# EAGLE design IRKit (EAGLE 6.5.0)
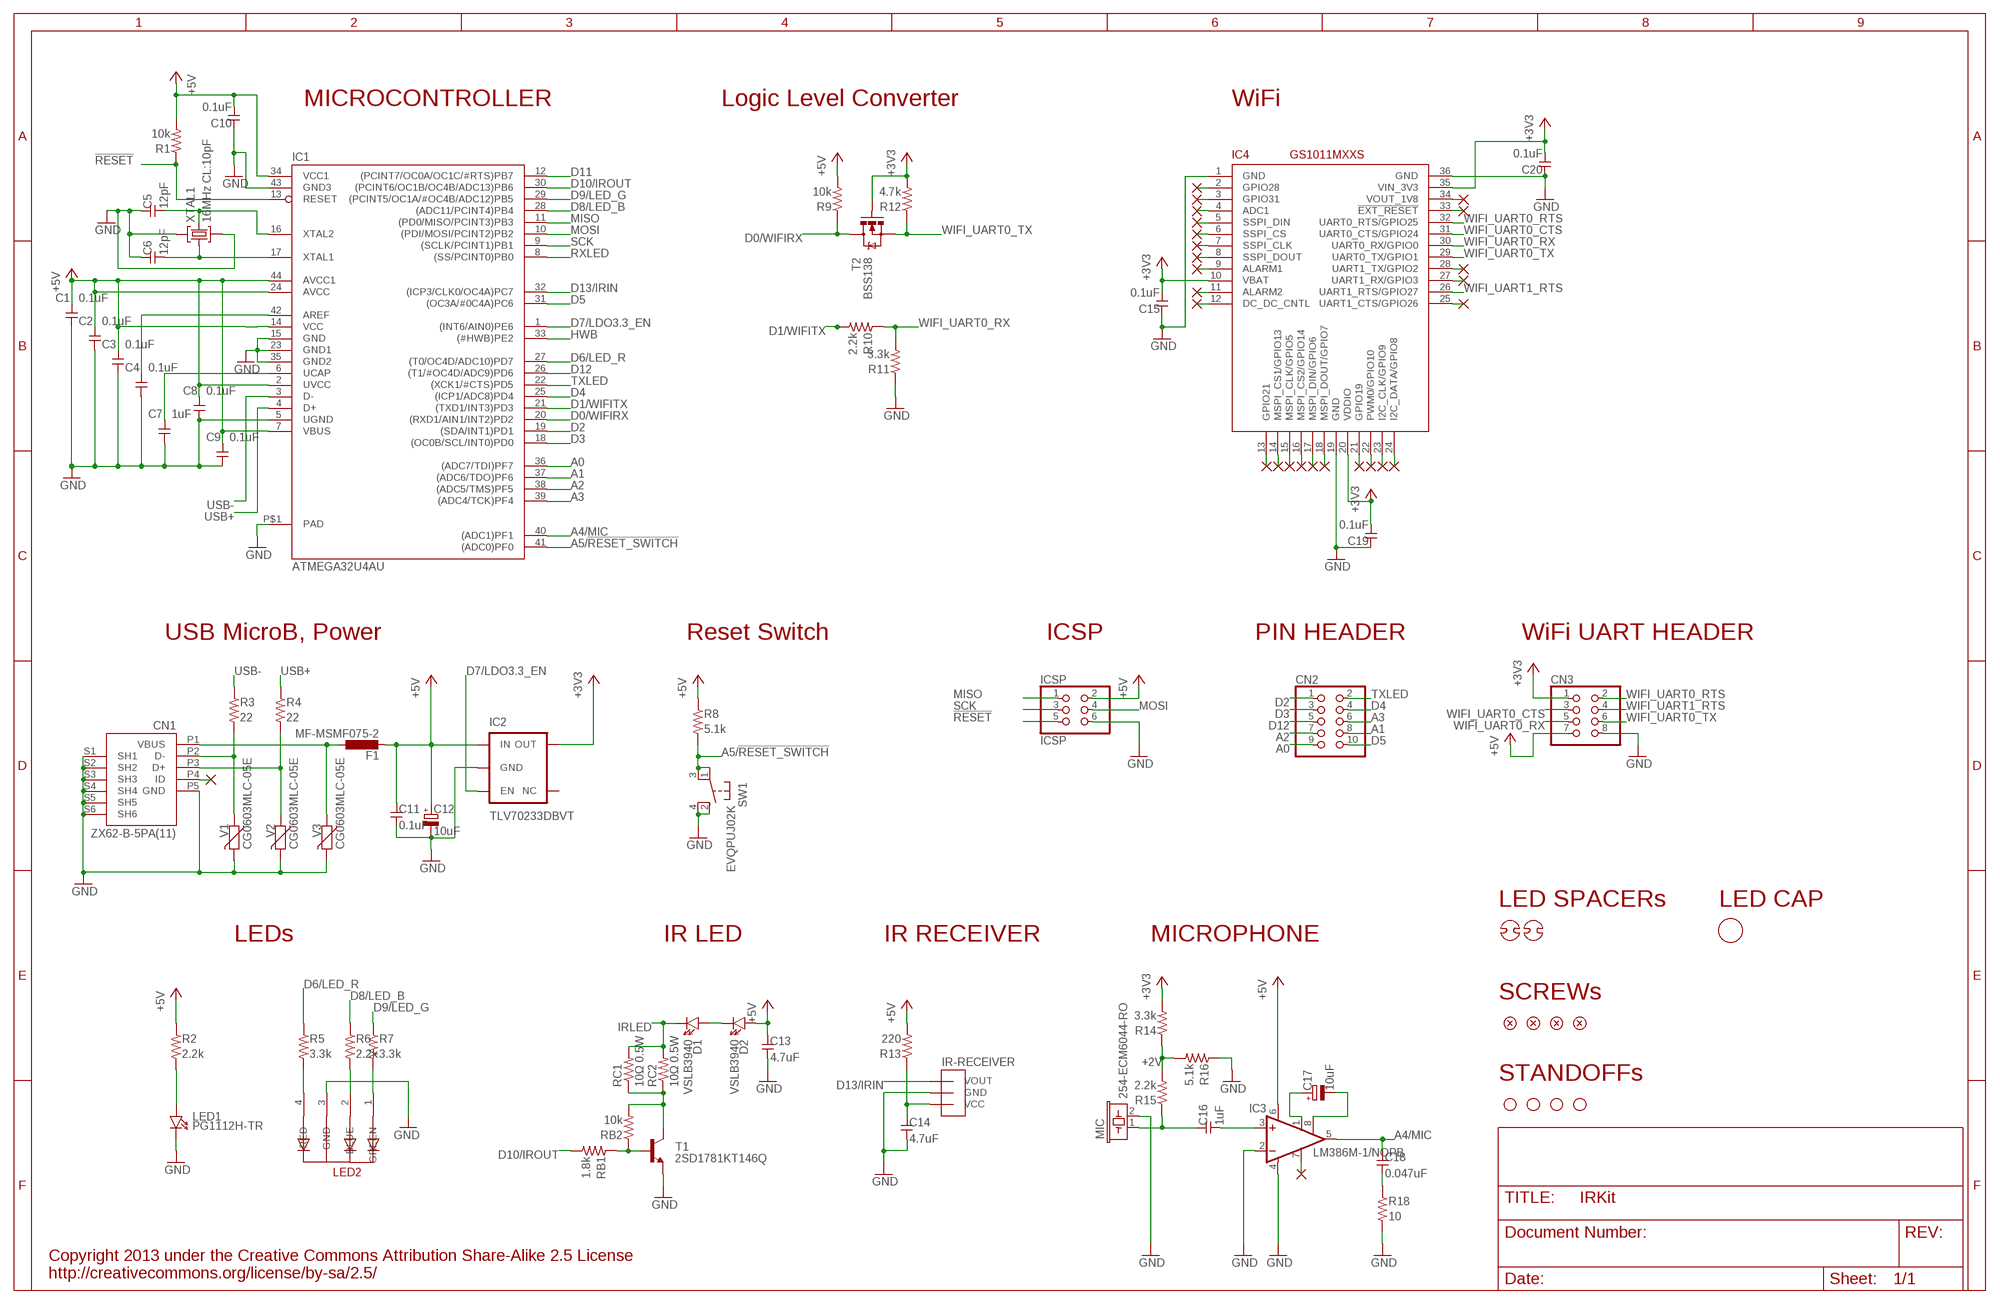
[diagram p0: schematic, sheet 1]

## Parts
C1  0.1uF  CAPACITOR2012  [SMD2012]
C2  0.1uF  CAPACITOR2012  [SMD2012]
C3  0.1uF  CAPACITOR2012  [SMD2012]
C4  0.1uF  CAPACITOR2012  [SMD2012]
C5  12pF  CAPACITOR2012  [SMD2012]
C6  12pF  CAPACITOR2012  [SMD2012]
C7  1uF  CAPACITOR2012  [SMD2012]
C8  0.1uF  CAPACITOR2012  [SMD2012]
C9  0.1uF  CAPACITOR2012  [SMD2012]
C10  0.1uF  CAPACITOR2012  [SMD2012]
C11  0.1uF  CAPACITOR2012  [SMD2012]
C12  10uF  CAPACITOR-POLPANASONIC_B  [PANASONIC_B]
C13  4.7uF  CAPACITOR2012  [SMD2012]
C14  4.7uF  CAPACITOR2012  [SMD2012]
C15  0.1uF  CAPACITOR2012  [SMD2012]
C16  1uF  CAPACITOR2012  [SMD2012]
C17  10uF  CAPACITOR-POLPANASONIC_B  [PANASONIC_B]
C18  0.047uF  CAPACITOR2012  [SMD2012]
C19  0.1uF  CAPACITOR2012  [SMD2012]
C20  0.1uF  CAPACITOR2012  [SMD2012]
CN1  ZX62-B-5PA(11)  USB-CONNECTORMICROB  [USB-MICROB]
CN2  PINHD-2X5  [2X05]
CN3  PINHD-2X4  [2X04]
D1  VSLB3940  LED-3MM  [LED3MM]
D2  VSLB3940  LED-3MM  [LED3MM]
F1  MF-MSMF075-2  L-EUL1812  [L1812]
IC1  ATMEGA32U4AU  [TQFP44-PAD]
IC2  TLV70233DBVT  TLV702XXSMD  [SOT23-5]
IC3  LM386M-1/NOPB  LM386M-1  [SO08]
IC4  GS1011MXXS  [GS1011MXXS]
ICSP  ICSP  PINHD-2X3  [2X03]
IR-RECEIVER  PL-IRM2161  [IR-RECEIVER]
LED1  PG1112H-TR  LED-2012  [LED2012]
LED2  5MMRGBLED  [LED5MMRGB]
LEDCAP1  LED-CAP  [LED-CAP]
MIC  254-ECM6044-RO  MICELECTRET_SMD  [MIC_SMD_4MM]
R1  10k  RESISTOR-US2012  [SMD2012]
R2  2.2k  RESISTOR-US2012  [SMD2012]
R3  22  RESISTOR-US2012  [SMD2012]
R4  22  RESISTOR-US2012  [SMD2012]
R5  3.3k  RESISTOR-US2012  [SMD2012]
R6  2.2k  RESISTOR-US2012  [SMD2012]
R7  3.3k  RESISTOR-US2012  [SMD2012]
R8  5.1k  RESISTOR-US2012  [SMD2012]
R9  10k  RESISTOR-US2012  [SMD2012]
R10  2.2k  RESISTOR-US2012  [SMD2012]
R11  3.3k  RESISTOR-US2012  [SMD2012]
R12  4.7k  RESISTOR-US2012  [SMD2012]
R13  220  RESISTOR-US2012  [SMD2012]
R14  3.3k  RESISTOR-US2012  [SMD2012]
R15  2.2k  RESISTOR-US2012  [SMD2012]
R16  5.1k  RESISTOR-US2012  [SMD2012]
R18  10  RESISTOR-US2012  [SMD2012]
RB1  1.8k  RESISTOR-US2012  [SMD2012]
RB2  10k  RESISTOR-US2012  [SMD2012]
RC1  10Ω 0.5W  R3225  [3225]
RC2  10Ω 0.5W  R3225  [3225]
SCREW1  flat-head M3 self-tapping  SCREW  [SCREW-M3]
SCREW2  flat-head M3 self-tapping  SCREW  [SCREW-M3]
SCREW3  flat-head M3 self-tapping  SCREW  [SCREW-M3]
SCREW4  flat-head M3 self-tapping  SCREW  [SCREW-M3]
SP1  LK-5  LED-SPACER-LK  [LED-SPACER-LK]
SP2  LK-5  LED-SPACER-LK  [LED-SPACER-LK]
STANDOFF1  STAND-OFF  [STAND-OFF]
STANDOFF2  STAND-OFF  [STAND-OFF]
STANDOFF3  STAND-OFF  [STAND-OFF]
STANDOFF4  STAND-OFF  [STAND-OFF]
SW1  EVQPUJ02K  TACTILE-SWITCHEVQPUJ02K  [TACTILE-SWITCH-EVQPUJ02K]
T1  2SD1781KT146Q  MMUN2211LT1-NPN-SC59-BEC  [SC59-BEC]
T2  BSS138  [SOT23]
V1  CG0603MLC-05E  VARISTORCN0603  [CT/CN0603]
V2  CG0603MLC-05E  VARISTORCN0603  [CT/CN0603]
V3  CG0603MLC-05E  VARISTORCN0603  [CT/CN0603]
XTAL1  16MHz CL:10pF  CRYSTAL-3.2-2.5  [CRYSTAL-3.2-2.5]

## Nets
!RESET: IC1.13(RESET) ICSP.5 R1.1
+2V: R14.1 R15.2 R16.2
+3V3 [3.3v]: C15.2 C19.2 C20.2 CN3.1 IC2.5(OUT) IC4.10(VBAT) IC4.20(VDDIO) IC4.35(VIN_3V3) R12.2 R14.2 T2.1(G)
+5V [power]: C1.2 C2.2 C3.2 C8.2 C9.2 C10.2 C11.1 C12.+ C13.1 CN3.7 D2.A F1.2 IC1.2(UVCC) IC1.7(VBUS) IC1.14(VCC) IC1.24(AVCC) IC1.34(VCC1) IC1.44(AVCC1) IC2.1(IN) IC3.6(VS) ICSP.2 R1.2 R2.1 R8.1 R9.2 R13.2
A0: CN2.9 IC1.36((ADC7/TDI)PF7)
A1: CN2.8 IC1.37((ADC6/TDO)PF6)
A2: CN2.7 IC1.38((ADC5/TMS)PF5)
A3: CN2.6 IC1.39((ADC4/TCK)PF4)
A4/MIC: C18.1 IC1.40((ADC1)PF1) IC3.5(OUT)
A5/!RESET_SWITCH: IC1.41((ADC0)PF0) R8.2 SW1.1(A) SW1.3(A)
AREF [power]: C4.2 IC1.42(AREF)
D0/WIFIRX: IC1.20((RXD1/AIN1/INT2)PD2) R9.1 T2.3(D)
D1/WIFITX: IC1.21((TXD1/INT3)PD3) R10.2
D2: CN2.1 IC1.19((SDA/INT1)PD1)
D3: CN2.3 IC1.18((OC0B/SCL/INT0)PD0)
D4: CN2.4 IC1.25((ICP1/ADC8)PD4)
D5: CN2.10 IC1.31((OC3A/#0C4A)PC6)
D6/LED_R: IC1.27((T0/OC4D/ADC10)PD7) R5.1
D7/LDO3.3_EN: IC1.1((INT6/AIN0)PE6) IC2.3(EN)
D8/LED_B: IC1.28((ADC11/PCINT4)PB4) R6.1
D9/LED_G: IC1.29((PCINT5/OC1A/#OC4B/ADC12)PB5) R7.1
D10/IROUT: IC1.30((PCINT6/OC1B/OC4B/ADC13)PB6) RB1.2
D11: IC1.12((PCINT7/OC0A/OC1C/#RTS)PB7)
D12: CN2.5 IC1.26((T1/#OC4D/ADC9)PD6)
D13/IRIN: IC1.32((ICP3/CLK0/OC4A)PC7) IR-RECEIVER.1(VOUT)
GND [gnd]: C1.1 C2.1 C3.1 C4.1 C5.1 C6.1 C7.1 C8.1 C9.1 C10.1 C11.2 C12.- C13.2 C14.2 C15.1 C19.1 C20.1 CN1.P5(GND) CN1.S1(SH1) CN1.S2(SH2) CN1.S3(SH3) CN1.S4(SH4) CN1.S5(SH5) CN1.S6(SH6) CN3.8 IC1.5(UGND) IC1.15(GND) IC1.23(GND1) IC1.35(GND2) IC1.43(GND3) IC1.P$1(PAD) IC2.2(GND) IC3.2(-IN) IC3.4(GND) IC4.1(GND) IC4.19(GND) IC4.36(GND) ICSP.6 IR-RECEIVER.2(GND) LED1.K LED2.3(GND) MIC.2 R11.1 R16.1 R18.2 SW1.2(B) SW1.4(B) T1.E V1.2 V2.2 V3.2 XTAL1.2(GND) XTAL1.4(GND)
HWB: IC1.33((#HWB)PE2)
IRLED [ir-power]: D1.K RC1.2 RC2.2
MICOUT: C16.1 MIC.1 R15.1
MISO: IC1.11((PD0/MISO/PCINT3)PB3) ICSP.1
MOSI: IC1.10((PDI/MOSI/PCINT2)PB2) ICSP.4
N$1: C17.- IC3.8(GAIN)
N$3: LED1.A R2.2
N$4: C16.2 IC3.3(+IN)
N$5: LED2.1(GREEN) R7.2
N$6: IC3.7(BYPASS)
N$8: C17.+ IC3.1(GAIN)
N$10: RB1.1 RB2.1 T1.B
N$11 [ir-power]: RB2.2 RC1.1 RC2.1 T1.C
N$14: C18.2 R18.1
N$16: C14.1 IR-RECEIVER.3(VCC) R13.1
N$17: LED2.2(BLUE) R6.2
N$18: IC4.2(GPIO28)
N$19: IC4.8(SSPI_DOUT)
N$20: IC4.9(ALARM1)
N$21: IC4.3(GPIO31)
N$22: IC4.4(ADC1)
N$23: IC4.5(SSPI_DIN)
N$24: IC4.6(SSPI_CS)
N$25: IC4.7(SSPI_CLK)
N$26: IC4.11(ALARM2)
N$27: IC4.12(DC_DC_CNTL)
N$28: IC4.13(GPIO21)
N$29: IC4.14(MSPI_CS1/GPIO13)
N$30: IC4.15(MSPI_CLK/GPIO5)
N$31: IC4.16(MSPI_CS2/GPIO14)
N$32: IC4.17(MSPI_DIN/GPIO6)
N$33: IC4.18(MSPI_DOUT/GPIO7)
N$34: IC4.21(GPIO19)
N$35: IC4.22(PWM0/GPIO10)
N$36: IC4.23(I2C_CLK/GPIO9)
N$37: IC4.24(I2C_DATA/GPIO8)
N$38: IC4.25(UART1_CTS/GPIO26)
N$39: IC4.27(UART1_RX/GPIO3)
N$40: IC4.28(UART1_TX/GPIO2)
N$41: LED2.4(RED) R5.2
N$43: IC4.34(VOUT_1V8)
N$44: IC4.33(!EXT_RESET)
N$48: CN1.P2(D-) R3.2 V1.1
N$51: CN1.P3(D+) R4.2 V2.1
N$52: CN1.P1(VBUS) F1.1 V3.1
N$58 [power]: D1.A D2.K
RXLED: IC1.8((SS/PCINT0)PB0)
SCK: IC1.9((SCLK/PCINT1)PB1) ICSP.3
TXLED: CN2.2 IC1.22((XCK1/#CTS)PD5)
UCAP: C7.2 IC1.6(UCAP)
USB+: IC1.4(D+) R4.1
USB-: IC1.3(D-) R3.1
USB-ID: CN1.P4(ID)
WIFI_UART0_CTS: CN3.3 IC4.31(UART0_CTS/GPIO24)
WIFI_UART0_RTS: CN3.2 IC4.32(UART0_RTS/GPIO25)
WIFI_UART0_RX: CN3.5 IC4.30(UART0_RX/GPIO0) R10.1 R11.2
WIFI_UART0_TX: CN3.6 IC4.29(UART0_TX/GPIO1) R12.1 T2.2(S)
WIFI_UART1_RTS: CN3.4 IC4.26(UART1_RTS/GPIO27)
XTAL1: C6.2 IC1.17(XTAL1) XTAL1.1(C1)
XTAL2: C5.2 IC1.16(XTAL2) XTAL1.3(C2)
Unconnected: IC2.4(NC)

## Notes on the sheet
- MICROCONTROLLER | Logic Level Converter | WiFi
- USB MicroB, Power | Reset Switch | ICSP | PIN HEADER | WiFi UART HEADER
- LED SPACERs | LED CAP
- LEDs | IR LED | IR RECEIVER | MICROPHONE
- SCREWs
- STANDOFFs
- Copyright 2013 under the Creative Commons Attribution Share-Alike 2.5 License
  http://creativecommons.org/license/by-sa/2.5/

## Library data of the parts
C1-C11 C13-C16 C18-C20 = my:CAPACITOR: Generic Capacitor
C12 C17 = my:CAPACITOR-POL: Generic Capacitor with Polarity
CN1 = my:USB-CONNECTOR
CN2 = my:PINHD-2X5: PIN HEADER
CN3 = my:PINHD-2X4: PIN HEADER
D1 D2 LED1 = my:LED: Through-hole LED
F1 = my:L-EU: INDUCTOR, European symbol
IC1 = my:ATMEGA32U4
IC2 = my:TLV702XX: TLV702xx http://www.tij.co.jp/jp/lit/ds/symlink/tlv70233.pdf http://www.ti.com/lit/ds/slvsag6b/slvsag6b.pdf 300-mA, Low-IQ, Low-Dropout Regulator
IC3 = my:LM386?-*: Low Voltage Audio Power Amplifier Source: http://cache.national.com/ds/LM/LM386.pdf
IC4 = my:GS1011MXXS
ICSP = my:PINHD-2X3: PIN HEADER
IR-RECEIVER = my:PL-IRM2161: PL-IRM2161-XD1 IR Receiver http://akizukidenshi.com/catalog/g/gI-06491/ http://akizukidenshi.com/download/ds/paralight/PL-IRM2161-XD1.pdf
LED2 = my:5MMRGBLED
LEDCAP1 = my:LED-CAP
MIC = my:MIC: Omni-directional electret condenser microphone.
R1-R16 R18 RB1 RB2 = my:RESISTOR-US: Generic Registor
RC1 RC2 = my:R: RESISTOR
SCREW1-SCREW4 = my:SCREW
SP1 SP2 = my:LED-SPACER
STANDOFF1-STANDOFF4 = my:STAND-OFF: #4 Stand Off
SW1 = my:TACTILE-SWITCH: TACTILE SWITCH
T1 = transistor:*-NPN-: NPN Transistror BF959 corrected 2008.03.06
T2 = my:BSS138
V1-V3 = my:VARISTOR: VARISTOR
XTAL1 = my:CRYSTAL-3.2-2.5

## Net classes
0 default: width 0.254 mm
1 power: width 0.406 mm
2 ir-power: width 0.813 mm
3 gnd: width 0.406 mm
4 3.3v: width 0.406 mm

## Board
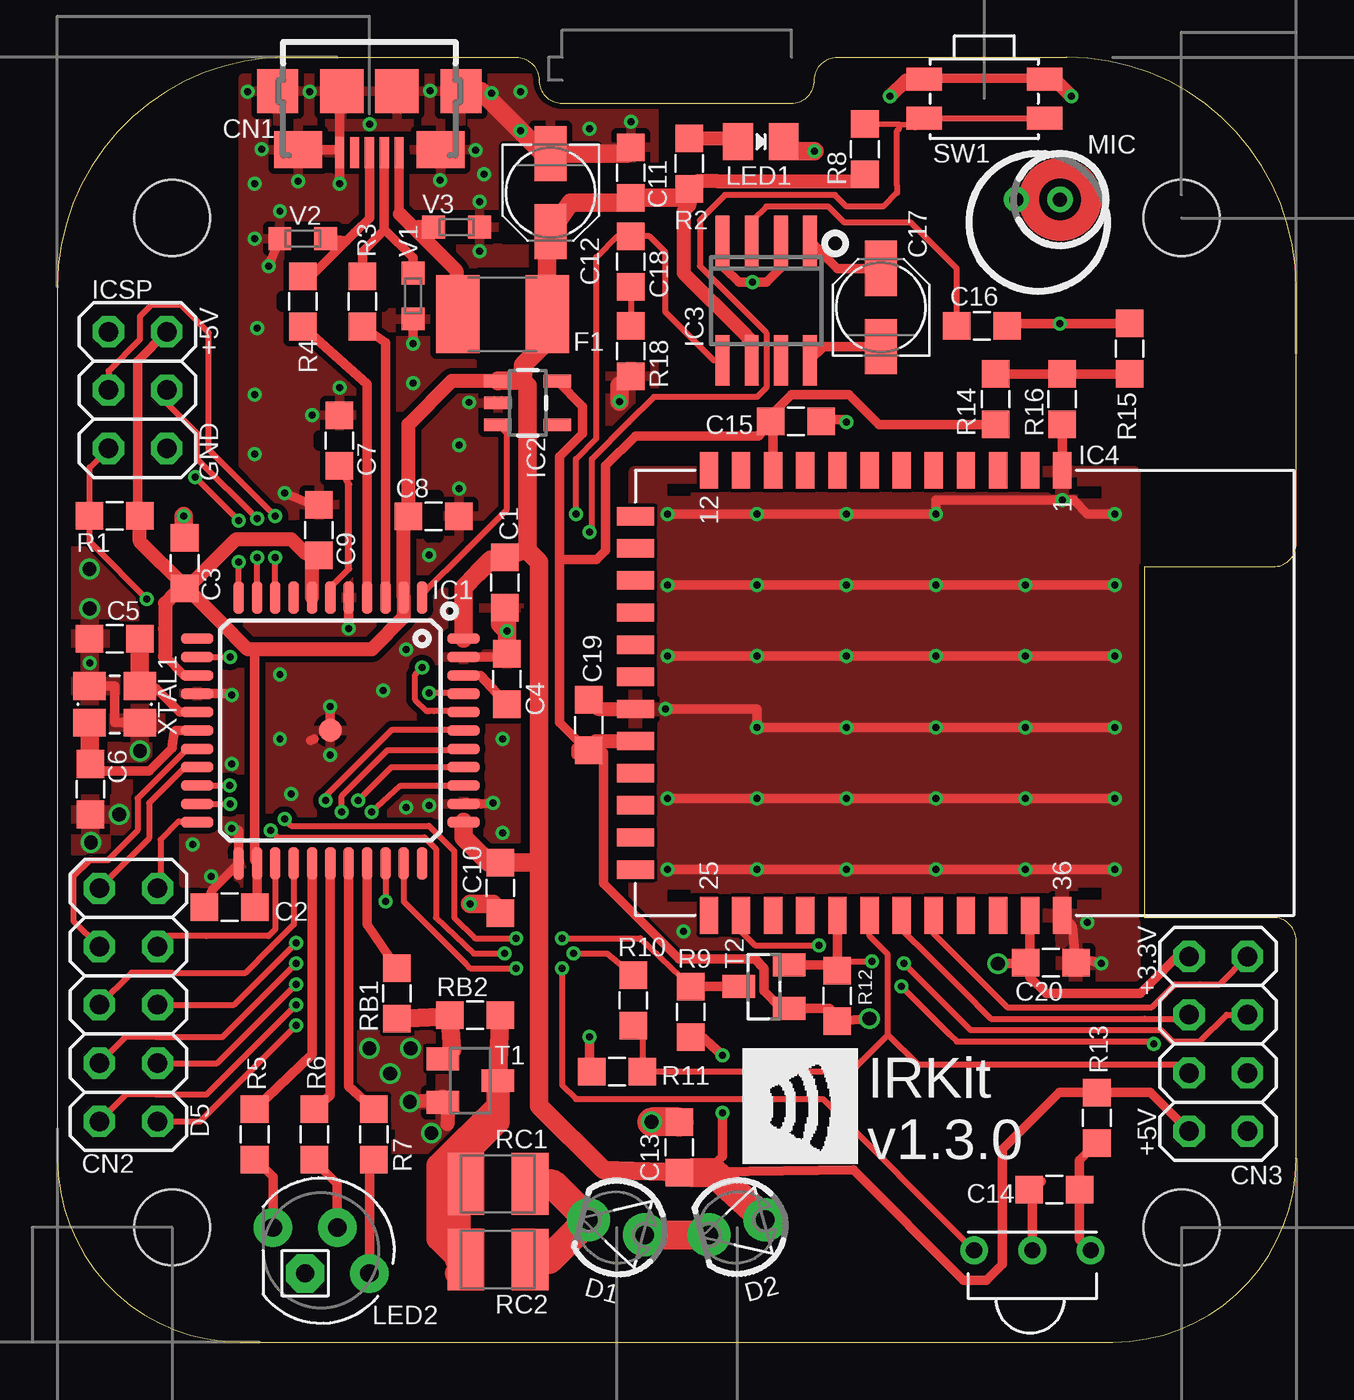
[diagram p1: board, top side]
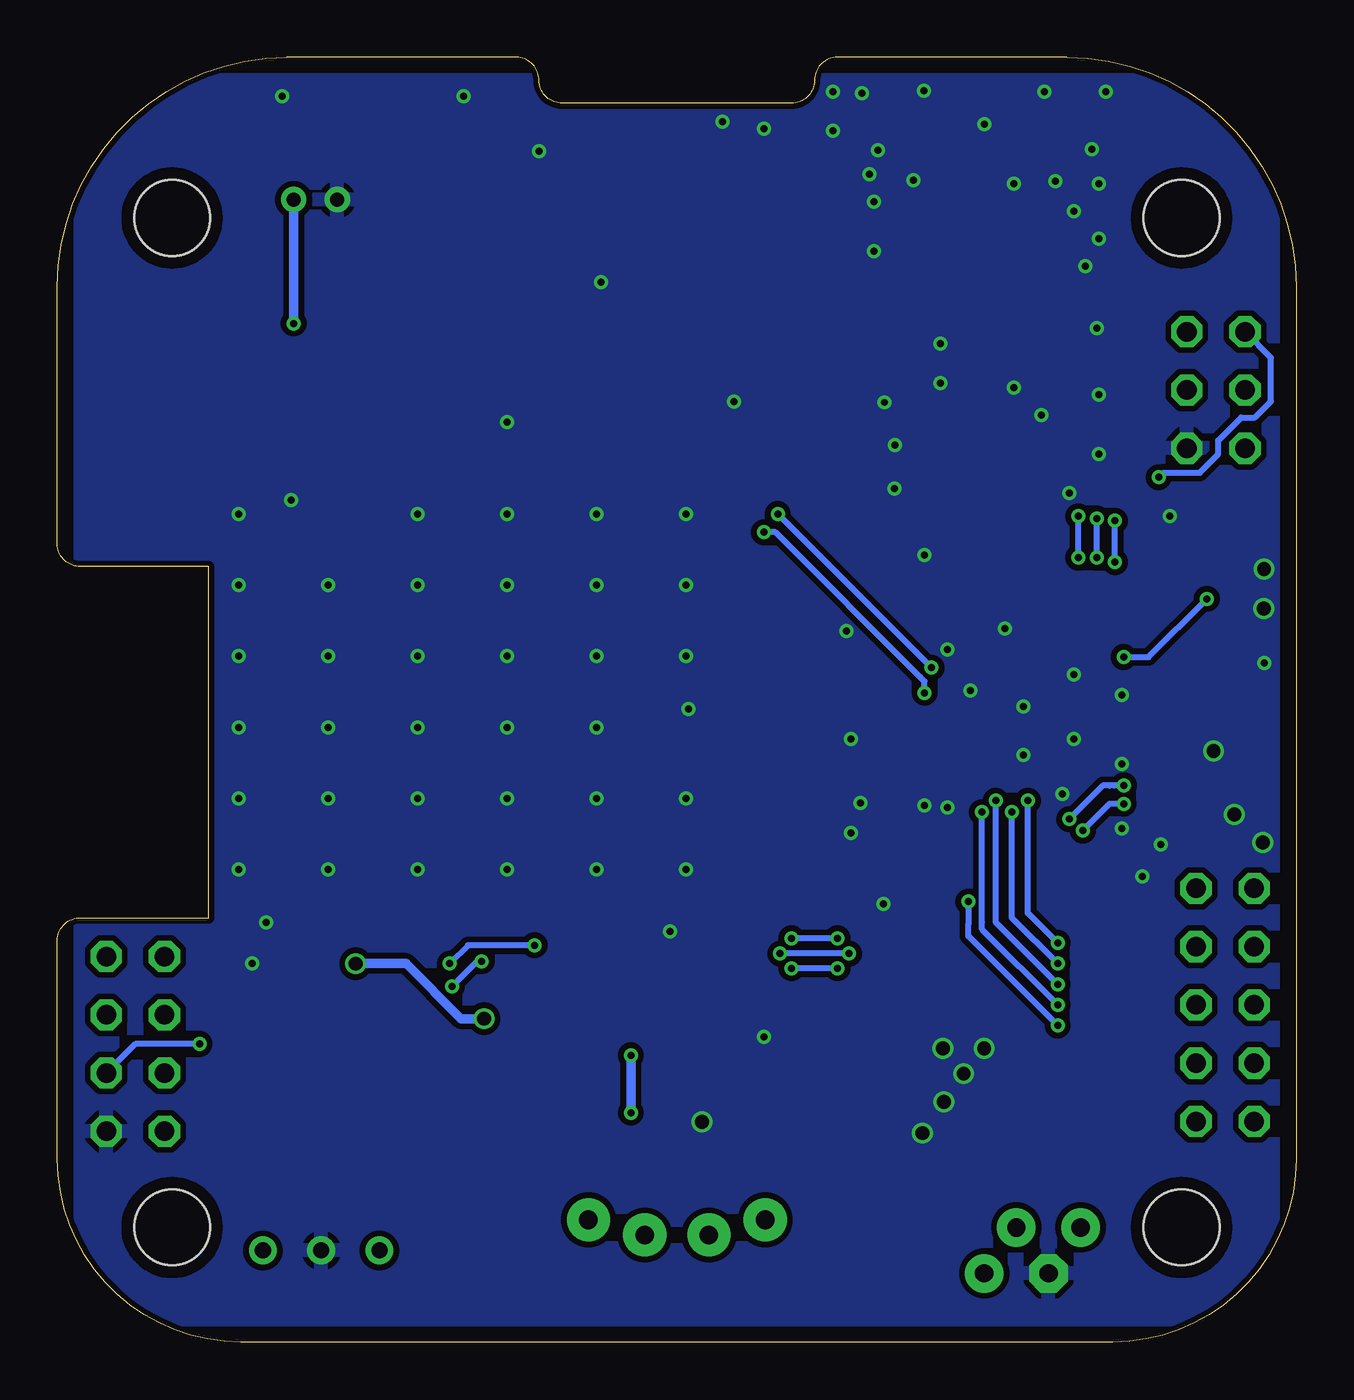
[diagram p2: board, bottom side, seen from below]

Size 54 x 56 mm. Coordinates in mm from the lower left corner, seen from the top.
Outline: 8,0 46,0 arc90 54,8 54,17.5 arc90 53,18.5 47.4,18.5 47.4,33.6 47.4,33.8 53,33.8 arc90 54,34.8 54,46 arc90 44,56 34,56 arc90 33,55 arc-90 32,54 22,54 arc-90 21,55 arc90 20,56 10,56 arc90 0,46 0,8 arc90 8,0
Copper layers (1*16): Top 0.035mm / dielectric 1.5mm / Bottom 0.035mm
Design rules "Fusion_eagle_rule_v1.1": minimum track width 6mil, minimum drill 12mil, track to track 6mil, track to pad 6mil, pad to pad 6mil, via to via 6mil, smd to smd 0mil, copper to edge 10mil, drill to drill 10mil, minimum pad ring 10mil, minimum via ring 6mil, stop-mask expansion 2mil, vias tented up to drill 100mil, thermal gap 10mil

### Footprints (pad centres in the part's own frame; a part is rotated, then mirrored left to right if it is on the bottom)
SMD2012 = smd 1.2 x 1.2: 1 -1.1,0; 2 1.1,0
PANASONIC_B = smd 2.4 x 1.4: + 1.7,0; - -1.7,0
USB-MICROB = smd 0.4 x 1.35: P1 -1.3,2.675; P2 -0.65,2.675; P3 0,2.675; P4 0.65,2.675; P5 1.3,2.675 | smd 1.8 x 1.9: S1 -4,0; S2 4,0 | smd 2.1 x 1.6: S3 -3.1,2.55; S4 3.1,2.55 | smd 1.9 x 1.9: S5 -1.2,0; S6 1.2,0
2X05 = drill 0.85 octagon: 1 -5.08,-1.27; 2 -5.08,1.27; 3 -2.54,-1.27; 4 -2.54,1.27; 5 0,-1.27; 6 0,1.27; 7 2.54,-1.27; 8 2.54,1.27; 9 5.08,-1.27; 10 5.08,1.27
2X04 = drill 0.85 octagon: 1 -3.81,-1.27; 2 -3.81,1.27; 3 -1.27,-1.27; 4 -1.27,1.27; 5 1.27,-1.27; 6 1.27,1.27; 7 3.81,-1.27; 8 3.81,1.27
LED3MM = drill 0.813 pad 1.88: A -1.27,0; K 1.27,0
L1812 = smd 1.9 x 3.4: 1 -1.95,0; 2 1.95,0
TQFP44-PAD = smd 1.4 x 0.45: 1 -5.8,4; 2 -5.8,3.2; 3 -5.8,2.4; 4 -5.8,1.6; 5 -5.8,0.8; 6 -5.8,0; 7 -5.8,-0.8; 8 -5.8,-1.6; 9 -5.8,-2.4; 10 -5.8,-3.2; 11 -5.8,-4; 23 5.8,-4; 24 5.8,-3.2; 25 5.8,-2.4; 26 5.8,-1.6; 27 5.8,-0.8; 28 5.8,0; 29 5.8,0.8; 30 5.8,1.6; 31 5.8,2.4; 32 5.8,3.2; 33 5.8,4 | smd 0.45 x 1.4: 12 -4,-5.8; 13 -3.2,-5.8; 14 -2.4,-5.8; 15 -1.6,-5.8; 16 -0.8,-5.8; 17 0,-5.8; 18 0.8,-5.8; 19 1.6,-5.8; 20 2.4,-5.8; 21 3.2,-5.8; 22 4,-5.8; 34 4,5.8; 35 3.2,5.8; 36 2.4,5.8; 37 1.6,5.8; 38 0.8,5.8; 39 0,5.8; 40 -0.8,5.8; 41 -1.6,5.8; 42 -2.4,5.8; 43 -3.2,5.8; 44 -4,5.8 | smd 1 x 1: P$1 0,0
SOT23-5 = smd 0.55 x 1.2: 1 -0.95,-1.3; 2 0,-1.3; 3 0.95,-1.3; 4 0.95,1.3; 5 -0.95,1.3
SO08 = smd 0.6 x 2.2: 1 -1.905,-2.6; 2 -0.635,-2.6; 3 0.635,-2.6; 4 1.905,-2.6; 5 1.905,2.6; 6 0.635,2.6; 7 -0.635,2.6; 8 -1.905,2.6
GS1011MXXS = smd 1.6 x 0.8: 1 0,18.6; 2 0,17.2; 3 0,15.8; 4 0,14.4; 5 0,13; 6 0,11.6; 7 0,10.2; 8 0,8.8; 9 0,7.4; 10 0,6; 11 0,4.6; 12 0,3.2; 25 19.4,3.2; 26 19.4,4.6; 27 19.4,6; 28 19.4,7.4; 29 19.4,8.8; 30 19.4,10.2; 31 19.4,11.6; 32 19.4,13; 33 19.4,14.4; 34 19.4,15.8; 35 19.4,17.2; 36 19.4,18.6 | smd 0.8 x 1.6: 13 2,0; 14 3.4,0; 15 4.8,0; 16 6.2,0; 17 7.6,0; 18 9,0; 19 10.4,0; 20 11.8,0; 21 13.2,0; 22 14.6,0; 23 16,0; 24 17.4,0
2X03 = drill 0.85 octagon: 1 -2.54,-1.27; 2 -2.54,1.27; 3 0,-1.27; 4 0,1.27; 5 2.54,-1.27; 6 2.54,1.27
IR-RECEIVER = drill 0.7: 1 -2.54,0; 2 0,0; 3 2.54,0
LED2012 = smd 1.3 x 1.6: A -1,0; K 1,0
LED5MMRGB = drill 0.8 pad 1.676: 1 2.1,-1; 2 0.7,1; 4 -2.1,1 | drill 0.8 pad 1.676 octagon: 3 -0.7,-1
MIC_SMD_4MM = drill 0.6: 1 1.9,0; 2 0,0
3225 = smd 1.6 x 2.7: 1 -1.4,0; 2 1.4,0
STAND-OFF = hole 3.302: 0,0
TACTILE-SWITCH-EVQPUJ02K = smd 1.55 x 1: 1 -2.625,-0.85; 2 -2.625,0.85; 3 2.625,-0.85; 4 2.625,0.85
SC59-BEC = smd 1 x 1.4: B -0.95,-1.2; C 0,1.2; E 0.95,-1.2
SOT23 = smd 1 x 1.4: 1 -0.95,-1.1; 2 0.95,-1.1; 3 0,1.1
CT/CN0603 = smd 1 x 1: 1 -1,0; 2 1,0
CRYSTAL-3.2-2.5 = smd 1.4 x 1.2: 1 -1.1,-0.8; 2 1.1,-0.8; 3 1.1,0.8; 4 -1.1,0.8

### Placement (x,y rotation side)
C1  19.5,33.1 90 top
C2  7.51,18.95 0 top
C3  5.55,33.95 270 top
C4  19.6,28.9 270 top
C5  2.5,30.66 0 top
C6  1.44,24.1 90 top
C7  12.3,39.3 270 top
C8  16.4,36 180 top
C9  11.4,35.4 270 top
C10  19.3,19.8 90 top
C11  25,50.97 90 top
C12  21.5,50.1 270 top
C13  27.1,8.5 90 top
C14  43.45,6.65 180 top
C15  32.2,40.14 180 top
C16  40.3,44.3 180 top
C17  35.9,45.1 90 top
C18  25,47.1 270 top
C19  23.16,26.9 270 top
C20  43.3,16.54 180 top
CN1  13.6,54.52 180 top
CN2  3.1,14.7 270 top
CN3  50.6,13 270 top
D1  24.38,5 165 top
D2  29.62,5 195 top
F1  19.4,44.8 0 top
IC1  11.9,26.66 270 top
IC2  20.5,40.94 270 top
IC3  30.9,45.4 180 top
IC4  25.2,38 270 top
ICSP  3.5,41.5 270 top
IR-RECEIVER  42.5,4 0 top
LED1  30.66,52.33 0 top
LED2  11.5,4 0 top
LEDCAP1  11.5,-0.7 0 top
MIC  41.8,49.8 0 top
R1  2.5,36.02 0 top
R2  27.55,51.38 90 top
R3  13.3,45.36 90 top
R4  10.7,45.36 90 top
R5  8.6,9.05 270 top
R6  11.2,9.05 270 top
R7  13.8,9.05 270 top
R8  35.2,52 90 top
R9  27.6,14.4 270 top
R10  25.1,14.9 90 top
R11  24.4,11.8 0 top
R12  34,15.1 270 top
R13  45.31,9.78 90 top
R14  40.9,41.1 270 top
R15  46.74,43.3 270 top
R16  43.8,41.1 90 top
R18  25,43.2 270 top
RB1  14.8,15.2 90 top
RB2  18.2,14.26 0 top
RC1  19.2,6.9 0 top
RC2  19.2,3.6 0 top
SCREW1  not placed on the board
SCREW2  not placed on the board
SCREW3  not placed on the board
SCREW4  not placed on the board
SP1  29.62,5 195 top
SP2  24.38,5 345 top
STANDOFF1  49,5 0 top
STANDOFF2  5,5 0 top
STANDOFF3  49,49 0 top
STANDOFF4  5,49 0 top
SW1  40.4,54.2 0 top
T1  18,11.4 270 top
T2  30.8,15.5 90 top
U$1  [IRKIT-LOGO]  29.9,7.8 0 top
V1  15.5,45.6 270 top
V2  10.7,48.1 180 top
V3  17.4,48.6 0 top
XTAL1  2.5,27.8 0 top

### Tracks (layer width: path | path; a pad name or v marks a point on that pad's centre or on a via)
!RESET  (via drill 0.3)
  Top 0.254: IC1.13 v7.53,29.86 | v3.9,32.4 1.6,34.7 1.4,34.9 R1.1 1.4,38.13 ICSP.5
  Bottom 0.254: v7.53,29.86 6.44,29.86 v3.9,32.4
+2V
  Top 0.406: R14.1 R16.2 R15.2
+3V3  (via drill 0.6)
  Top 0.406: IC4.35 42.4,16.8 | 42.4,16.8 42.4,16.74 | C19.2 22.6,25.6 22.6,25.7 22.6,25.9 | C19.2 23,25.9 21.9,27 21.9,29.3 21.9,34.1 | 31.2,40.1 IC4.10 | 31.2,40.1 C15.2 30.56,39.5 25.2,39.5 23.9,38.2 23.9,34.5 23.5,34.1 21.9,34.1 | 31.9,14.8 T2.1 | C19.2 23.46,26.2 | IC4.20 23.3,26.2 23.8,25.7 23.8,20 27.1,16.7 30.1,16.7 30.4,16.7 30.8,16.3 30.8,15.3 31.55,14.55 T2.1 | C20.2 42.4,16.44 42.4,15.9 43.1,15.2 47,15.2 47.2,15.2 48.2,16.2 48.81,16.81 CN3.1 | 42.4,16.8 42.3,16.8 C20.2 | T2.1 33.65,14.55 R12.2 v35.4,14.1 | v41,16.5 42.26,16.5 C20.2 | 31.2,40.1 31.2,40.5 32,41.3 34.5,41.3 35.8,40 36,40 R14.2 | 21.9,34.1 21.9,38.6 22.9,39.6 22.9,40.5 22.9,40.79 IC2.5
  Top 0.61: 23,25.9 C19.2 | 23.46,26.2 IC4.20
  Bottom 0.406: v35.4,14.1 36.4,14.1 38.8,16.5 v41,16.5
+5V  (via drill 0.3)
  Top 0.406: C2.2 8.7,19.41 IC1.24 8.6,21 8.6,29.9 8.6,30.2 | ICSP.2 3.5,42.77 3.5,38.3 3.5,36.62 R1.2 | 5.1,32.6 5.1,32.7 C3.2 | 4.7,29.9 5.54,29.06 IC1.14 | 21.35,46.73 21.35,47.9 | v29,10 29,8.1 28.4,7.5 27.7,7.4 | v29,12.5 28,13.4 R9.2 | C13.1 34.7,7.5 39.5,2.7 40.5,2.7 41.2,3.4 41.2,8.4 43.68,10.88 R13.2 | 44.99,10.7 R13.2 | R13.2 47.64,10.88 CN3.7 | C10.2 19.4,20.9 | 27.3,49.3 27.3,49.5 27.15,49.87
  Top 0.61: 4.8,43.7 ICSP.2 | IC1.7 11.1,34.1 C9.2 10.8,34.4 10.2,35 7.8,35 5.75,32.95 5.55,32.95 | 5.55,32.95 7.1,31.4 8.3,30.2 8.6,30.2 13.7,30.2 15.1,31.6 IC1.2 15.1,35.9 C8.2 15.3,40 17.2,41.9 19.19,41.9 IC2.1 | 5.55,32.95 C3.2 | 5.1,32.6 4.7,32.2 4.7,31.1 4.7,29.9 | CN3.7 | 5.55,32.95 3.6,34.9 R1.2 | R8.1 35.2,50.6 28.8,50.6 27.88,50.6 R2.1 27.55,49.55 27.3,49.3 27.3,46.6 29.8,44.1 30.27,43.63 IC3.6
  Top 0.813: 20.5,34.5 20.5,34.55 20.5,41.7 20.3,41.9 | 20.5,34.5 21,34 21,20.9 | 20.5,34.5 20.3,34.5 C1.2 18.9,34.1 18.3,33.5 | 18.6,33.8 18.3,33.5 | 18.3,33.5 17.7,32.9 IC1.44 | 19.4,20.9 21,20.9 | 21,20.9 21,10.3 23.8,7.5 C13.1 27.7,7.4 | IC1.34 17.7,22 18.8,20.9 C10.2 | 27.15,49.87 C11.1 24.7,49.67 22.37,49.67 C12.+ 21.35,48.55 21.35,47.9 F1.2 21.35,43.62 20.3,42.58 20.3,41.9 | 20.3,41.9 19.21,41.9 IC2.1
  Top 1.27: 27.7,7.4 28.58,7.4 D2.A
  Bottom 0.406: v29,10 v29,12.5
A0  (via drill 0.3)
  Top 0.254: IC1.36 15.06,24.26 14.96,24.26 v13.7,23.1 | CN2.9 3.01,10.8 4.3,10.8 6.5,10.8 v10.4,14.7
  Bottom 0.254: v13.7,23.1 13.7,18.3 13.7,18 v10.4,14.7
A1  (via drill 0.3)
  Top 0.254: 17.7,25 IC1.37 14.56,25.06 v13.1,23.6 | CN2.8 6.96,12.16 v10.4,15.6
  Bottom 0.254: v10.4,15.6 13.1,18.3 v13.1,23.6
A2  (via drill 0.3)
  Top 0.254: CN2.7 2.97,13.3 4.3,13.3 4.4,13.3 7.2,13.3 v10.4,16.5 | 17.7,25.8 IC1.38 17.64,25.8 15.1,25.8 | v12.4,23.1 12.4,23.8 14.4,25.8 15.1,25.8 | 14.5,25.8 15.1,25.8
  Bottom 0.254: v12.4,23.1 12.4,18.8 12.4,18.5 v10.4,16.5
A3  (via drill 0.3)
  Top 0.254: v11.7,23.6 11.7,23.8 14.6,26.7 17.66,26.7 IC1.39 | CN2.6 7.7,14.7 v10.4,17.4
  Bottom 0.254: v11.7,23.6 11.7,18.9 11.7,18.7 v10.4,17.4
A4/MIC  (via drill 0.3)
  Top 0.254: 17.7,27.4 IC1.40 17.66,27.5 16.4,27.5 16.2,27.5 16.1,27.5 15.6,28 15.6,29.1 v15.9,29.4 | IC3.5 28.6,42.8 26.5,44.9 26.5,47.5 25.8,48.2 C18.1 24.4,48.2 23.5,47.3 23.5,46.5 23.5,39.4 22.6,38.5 v22.6,36.1
  Bottom 0.254: v15.9,29.4 v22.6,36.1
A5/!RESET_SWITCH  (via drill 0.3)
  Top 0.254: SW1.3 SW1.1 37.5,53.08 36.7,53.09 | IC1.41 17.66,28.3 v16.2,28.3 | v23.2,35.3 23.3,35.4 23.3,38.5 24.9,40.1 26,41.2 26.1,41.2 30.5,41.2 30.9,41.6 30.9,44 28,46.9 28,48.9 29.1,50 33.9,50 34.4,49.5 34.7,49.5 36,49.5 36.6,50.1 36.6,50.4 36.6,52.8 36.7,52.9 36.7,53 36.7,53.09 | R8.2 36.7,53.09
  Top 0.305: 37.4,52.98 SW1.1
  Bottom 0.254: v23.2,35.3 22.7,35.3 16.4,29 16.2,28.8 v16.2,28.3
AREF
  Top 0.406: IC1.42 18.44,29.06 C4.2
D0/WIFIRX  (via drill 0.3)
  Top 0.254: IC1.20 v7.51,24.26 | v20,17.6 18.2,17.6 17.3,18.5 17.3,21.4 16.2,22.5 10.2,22.5 v9.9,22.8 | v22,17.6 25.4,17.6 R9.1
  Top 0.406: R9.1 T2.3
  Bottom 0.254: v20,17.6 v22,17.6 | v7.51,24.26 7.74,24.26 7.94,24.26 8.14,24.26 8.44,24.26 v9.9,22.8
D1/WIFITX  (via drill 0.3)
  Top 0.254: IC1.21 v7.53,23.46 | v19.49,16.94 18.15,16.94 16.5,18.5 16.5,21.5 16,22 9.6,22 9.5,22.1 v9.3,22.3 | v22.5,16.94 23.96,16.94 R10.2
  Bottom 0.254: v19.49,16.94 v22.5,16.94 | v7.53,23.46 8.14,23.46 v9.3,22.3
D2
  Top 0.254: IC1.19 5.56,25.06 4,23.5 4,21.95 CN2.1
D3
  Top 0.254: IC1.18 5.66,25.86 3.5,23.7 3.5,22.3 2.2,21 1.4,21 0.7,20.3 0.7,18.37 CN2.3
D4
  Top 0.254: IC1.25 9.5,18 9.2,17.7 6.5,17.7 4.83,17.7 CN2.4 4.4,17.2
D5  (via drill 0.3)
  Top 0.254: IC1.31 v14.3,19.2 | CN2.10 6.22,9.62 v10.4,13.8
  Bottom 0.254: v14.3,19.2 14.3,18.2 14.3,17.7 v10.4,13.8
D6/LED_R
  Top 0.406: IC1.27 11.1,12.55 R5.1
D7/LDO3.3_EN
  Top 0.254: 19.6,40.09 IC2.3 19.6,39.59 19.6,36.3 17.9,34.6 15.9,32.6 IC1.1
D8/LED_B
  Top 0.406: IC1.28 11.9,10.75 R6.1
D9/LED_G
  Top 0.254: 13.8,10.1 R7.1
  Top 0.406: IC1.29 12.7,11.15 R7.1
D10/IROUT
  Top 0.406: IC1.30 13.5,18.2 RB1.2
D12
  Top 0.254: IC1.26 10.3,18.2 9.3,17.2 8.2,16.1 5,16.1 3.23,16.1 CN2.5
D13/IRIN  (via drill 0.3)
  Top 0.254: IC1.32 15.1,19.2 17.8,16.5 18,16.3 v20,16.3 | v22,16.3 22,11.2 22.6,10.6 32.1,10.6 33.36,10.6 IR-RECEIVER.1
  Bottom 0.254: v20,16.3 v22,16.3
GND  (via drill 0.3, 0.6)
  Top 0.406: IC1.P$1 v11.9,27.7 | v45.5,16.5 44.29,16.8 C20.1 44.25,18.15 IC4.36 | IC1.5 v12.7,31.1 | C2.1 6.76,19.73 IC1.23 7.9,22.3 | v7.6,28.2 7.34,28.26 6.24,28.26 6.1,28.3 | 6.1,28.3 IC1.15 | 6.1,28.3 IC1.15 | 6.1,28.3 IC1.15 | C12.- 21.3,51.7 | 24.9,52 C11.2 25.2,52 | C6.1 1.5,23.3 C6.1 | v19,23.5 18.46,23.46 18.3,23.5 17.7,23.5 IC1.35 | C9.1 11.1,36.5 v9.9,37 | V1.2 v15.5,43.52 | V2.2 v9.2,46.9 | 19.46,29.86 IC1.43 | C6.1 1.1,23.2 C6.1 | 5.5,35 C3.1 | SW1.4 42.8,55.1 37.6,55.1 SW1.2 37.4,55 | v46.1,36.1 44.9,36.1 44.3,36.7 v43.8,36.7 43.6,36.7 38.3,36.7 38.3,36.3 v38.3,36.1 34.6,36.1 v34.4,36.1 30.7,36.1 v30.5,36.1 v26.6,36.1 | v26.6,33 v30.5,33 30.7,33 v34.4,33 34.6,33 v38.3,33 38.5,33 v42.2,33 42.4,33 v46.1,33 | v26.6,29.9 v30.5,29.9 30.7,29.9 v34.4,29.9 34.6,29.9 v38.3,29.9 38.5,29.9 v42.2,29.9 42.4,29.9 v46.1,29.9 | v26.5,27.6 30.5,27.6 v30.5,26.8 30.7,26.8 v34.4,26.8 34.6,26.8 v38.3,26.8 38.5,26.8 v42.2,26.8 42.4,26.8 v46.1,26.8 | v26.6,23.7 v30.5,23.7 30.7,23.7 v34.4,23.7 34.6,23.7 v38.3,23.7 38.5,23.7 v42.2,23.7 42.4,23.7 v46.1,23.7 | v26.6,20.6 v30.5,20.6 30.7,20.6 v34.4,20.6 34.6,20.6 v38.3,20.6 38.5,20.6 v42.2,20.6 42.4,20.6 v46.1,20.6 | 43.8,40.2 R16.1 IC4.1 | C15.1 33.2,40.2 34.3,40.2 v34.4,40.1 | CN1.S6 12.8,54.4 CN1.S6 | IR-RECEIVER.2 42.5,6.6 42.9,7 C14.2 | R11.1 23.2,12.1 v23.2,13.3 | LED1.K 31.89,51.9 | XTAL1.4 2.5,28.6 2.5,27 XTAL1.2 | CN1.P5 v12.3,50.5 | CN1.S4 12.3,51.98 CN1.P5 | CN1.S6 12.3,54.52 CN1.P5 | IC3.4 | IC3.4 29,47.8 29.1,47.7 29.1,46.8 29.7,46.2 v30.3,46.2 30.9,46.2 31.5,46.8 31.5,48 IC3.2 | IC4.19 | 11.2,26.3 11.04,26.23 11.2,26.3
  Top 0.61: 37.4,55 37,55 v36.3,54.3 | SW1.4 43.45,55.05 v44.2,54.3 | T1.E 17,10.45 17,9.5 | v15.36,10.47 16.8,10.6 | C19.1 23.56,27.6 IC4.19
  Top 0.813: 19.46,29.86 C4.1 v19.6,31 | C1.1 19.6,31.8 v19.6,31 | 21.3,51.7 18.48,54.52 CN1.S1 | 25.2,52 25.1,52.1 | 19.3,31.3 v19.6,31 | v18,19.1 19,19.1 C10.1 | 31.89,51.9 v33,51.9 | R18.2 24.5,41.7 v24.5,41 | C12.- 24.82,51.8 C11.2 | 16.8,10.6 T1.E | 5.5,35 v5.5,36
  Top 1.27: C13.2 v25.9,9.6
  other vias: 7.6,22.4 2.7,23 11.1,40.4 1.4,33.7 1.41,31.98 1.46,21.77 16.2,23.4 9.7,29.1 9.7,26.3 11.9,25.6 14.2,28.4 8.6,38.7 12.3,41.6 10.5,50.6 8.3,54.5 8.6,41.3 8.7,44.2 17.51,37.2 7.6,25.2 16.69,50.64 18.4,47.55 18.93,54.44 8.6,48.1 15.5,41.8 5.9,21.7 6.7,20.3 17.5,39.1 13.6,53.09 16.24,54.55 18.23,51.96 10.99,54.5 8.9,52 19.4,26.3 19.4,22.2 10.2,23.9 15.2,23.3 13.6,12.8 20.2,54.5 20.2,52.8 25,53.2 23.2,52.9 18.4,49.7 44.9,18.3 17.95,40.96 15.4,12.8 15.2,30.2 9.7,49.3 8.6,50.5 18.6,50.9 16.3,9.11 14.5,11.7 3.6,25.76 1.4,29.6 27.3,17.9 16.21,34.3
  pour Bottom (isolate 0.254): 1,1 1,55 53,55 53,1
  pour Top: 1,35.3 4.3,35.3 4.3,21.1 1,21.1
  pour Top (isolate 0.254): 5.5,33.1 20,33.1 20,20 5.5,20
  pour Top (isolate 0.254): 26,32.2 8.1,32.2 8.1,55.1 26,55.1
  pour Top: 25.2,37.9 46.9,37.9 46.9,16 25.2,16
  pour Top: 12.9,13.3 17.1,13.3 17.2,8.5 13,8.5
IRLED
  Top 1.27: RC1.2 21.58,6.9 D1.K 21.42,3.6 RC2.2
MICOUT  (via drill 0.3)
  Top 0.406: R15.1 v43.7,44.4 41.5,44.4 C16.1
  Bottom 0.406: MIC.1 v43.7,44.4
MISO  (via drill 0.3)
  Top 0.254: IC1.11 v7.9,34 | v7.9,35.8 v6,37.7
  Bottom 0.254: ICSP.1 1.1,42.91 1.1,41 1.8,40.3 2.4,40.3 3.4,39.3 3.4,38.7 4.2,37.9 5.8,37.9 v6,37.7 | v7.9,34 v7.9,35.8
MOSI  (via drill 0.3)
  Top 0.254: IC1.10 v8.7,34.2 | ICSP.4 4.77,40.93 6.1,39.6 6.1,38.5 v8.7,35.9
  Bottom 0.254: v8.7,34.2 v8.7,35.9
N$1
  Top 0.406: C17.- 33.41,43.4 IC3.8
N$3
  Top 0.61: R2.2 29.51,52.48 LED1.A
N$4
  Top 0.254: C16.2 39.2,46.8 37.2,48.8 34.3,48.8 33.6,49.5 30.9,49.5 30.3,48.9 30.3,48.03 IC3.3
N$5
  Top 0.254: 13.6,7.8 13.8,8 R7.2 13.6,7.7
  Top 0.406: LED2.1 13.6,7.7
N$8
  Top 0.406: C17.+ 34.01,46.8 IC3.1
N$10
  Top 0.813: RB1.1 17.14,14.2 RB2.1 17.2,12.75 T1.B
N$11
  Top 0.813: RB2.2 T1.C
  Top 1.016: RC1.1 17.5,7.9 | 17.5,7.9 17.5,8 17.5,7.9 | T1.C 19.2,10.4 19.2,10.3 | RC2.1 17.4,3.6 17.4,3.7 16.6,4.5 16.6,7.7 19.2,10.3 | 17.5,7.9 17.5,3.1 17.4,3 | 19.2,10.3 19.2,9.6 17.5,7.9
N$14
  Top 0.254: C18.2 R18.1
N$16
  Top 0.406: IR-RECEIVER.3 44.55,4.49 C14.1 44.55,7.92 R13.1
N$17
  Top 0.254: 11.2,8 R6.2 11.2,7.9
  Top 0.406: 11.2,7.9 12.2,6.9 LED2.2
N$41
  Top 0.254: 8.6,8 R5.2 | 9.4,7.1 9.4,7.2
  Top 0.406: 9.4,7.2 8.6,8 | LED2.4 9.4,7.1
N$48
  Top 0.406: R3.2 13.3,47.54 14.26,48.5 | 14.26,48.5 15.5,47.26 V1.1 | 14.26,48.5 14.25,48.5 CN1.P2
N$51
  Top 0.254: R4.2 10.7,46.6 11,46.6 11.16,46.56
  Top 0.406: 12.95,48.35 13.6,49 CN1.P3 | 12.95,48.35 11.16,46.56 | V2.1 12.6,48 12.95,48.35
N$52
  Top 0.254: F1.1 17.5,45.5 17.4,45.5
  Top 0.406: 14.92,49.18 14.9,49.18 CN1.P1
  Top 0.61: 17.4,44.7 17.4,45.5 17.4,46.7 16,48.1 15.75,48.35 | 14.92,49.18 15.75,48.35 | V3.1 15.75,48.6 15.75,48.35
N$58
  Top 1.27: D1.A D2.K
SCK  (via drill 0.3)
  Top 0.254: IC1.9 v9.5,34.2 | ICSP.3 2.23,42.33 3.6,43.7 3.6,44.7 4.1,45.2 5.4,45.2 6.6,44 6.6,38.9 v9.5,36
  Bottom 0.254: v9.5,34.2 v9.5,36
TXLED
  Top 0.254: CN2.2 4.5,19.91 4.5,21.9 5.26,22.66 5.3,22.7 6.1,22.7 IC1.22
UCAP
  Top 0.254: IC1.6 11.9,32.9 12.7,33.7
  Top 0.305: 12.7,33.7 12.7,37.4 C7.2
USB+
  Top 0.406: IC1.4 13.5,41.76 R4.1
USB-
  Top 0.406: IC1.3 14.3,43.56 R3.1
WIFI_UART0_CTS
  Top 0.254: IC4.31 36.8,18 38,16.8 39.45,15.35 | 39.1,15.7 39.45,15.35 | 39.45,15.35 40.7,14.1 47.4,14.1 49.16,14.1 CN3.3
WIFI_UART0_RTS
  Top 0.254: IC4.32 38.2,17.8 40.6,15.4 | 40.2,15.8 40.6,15.4 | 40.6,15.4 41.4,14.6 47.7,14.6 48.7,15.6 49.8,15.6 50.66,15.6 CN3.2
WIFI_UART0_RX
  Top 0.254: CN3.5 48.96,12.1 43.7,12.1 37.5,12.1 36.2,13.4 | 36.2,13.4 36.2,16.9 35.4,17.7 IC4.30 | 36.2,13.4 34.7,11.9 34.6,11.8 R11.2 25.5,13.8 R10.1
WIFI_UART0_TX  (via drill 0.3)
  Top 0.254: 34.4,16.6 v35.5,16.6 | v47.8,13 47.7,13.1 39.2,13.1 38.9,13.4 v36.8,15.5
  Top 0.406: T2.2 33.75,16.45 R12.1 | R12.1 IC4.29 | R12.1 34.4,16.6
  Bottom 0.254: v35.5,16.6 35.7,16.6 v36.8,15.5 | v47.8,13 50.6,13 CN3.6
WIFI_UART1_RTS  (via drill 0.3)
  Top 0.254: IC4.26 29.8,17.9 30.4,17.3 v33.2,17.3 | 39.9,13.6 40.2,13.6 | 40.2,13.6 48.1,13.6 48.6,13.1 49.8,13.1 50.97,14.27 CN3.4 | v36.9,16.5 39.8,13.6 40.2,13.6
  Bottom 0.254: v33.2,17.3 36.1,17.3 v36.9,16.5
XTAL1
  Top 0.406: IC1.17 5.16,26.66 5.1,26.6 5,26 5,25.9 4,24.9 1.94,24.9 C6.2 1.74,25.1
  Top 0.813: XTAL1.1 1.4,25.44 C6.2
XTAL2
  Top 0.406: IC1.16 5.34,27.46 4.3,28.5 3.8,28.5 XTAL1.3
  Top 0.813: C5.2 3.6,28.7 XTAL1.3

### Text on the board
tPlace: +5V | GND | +3.3V | D5 | IRKit / v1.3.0 | +5V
